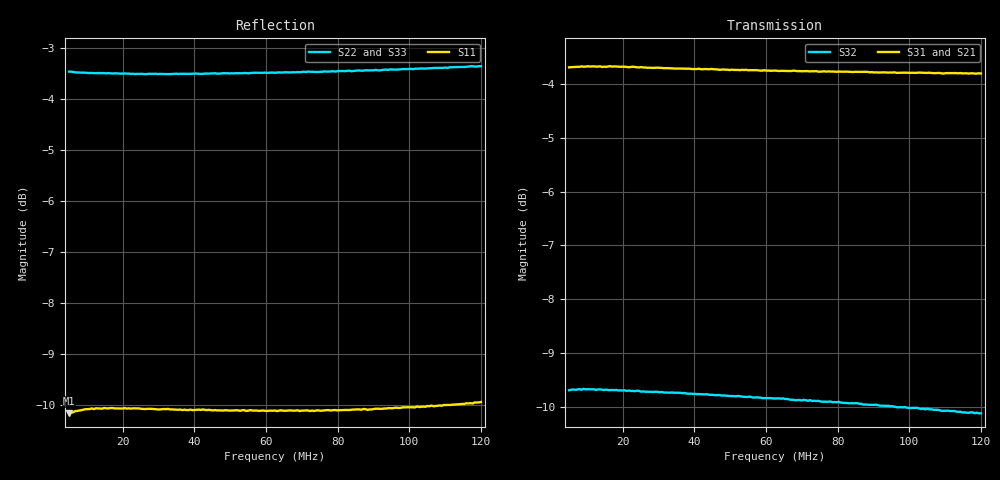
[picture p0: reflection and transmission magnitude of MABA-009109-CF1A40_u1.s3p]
#	MHz	S	RI	R	75
!FREQ	R1	I1	R2	I2	R3	I3
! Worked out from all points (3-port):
!   201 points, 5 MHz to 120 MHz, reference 75 ohm
!   strongest paths, dB at 5 MHz, 33.75 MHz, 62.5 MHz, 91.25 MHz, 120 MHz:
!     S31: -3.7, -3.7, -3.8, -3.8, -3.8
!     S21: -3.7, -3.7, -3.8, -4.0, -4.1
!     S32: -9.7, -9.7, -9.8, -10.0, -10.1
!   lowest |S11| = -10.2 dB at 5 MHz (marker M1), VSWR 1.90, Z = 142 + j2.55 ohm
!   |S11| at or under -10 dB: start of sweep to 109.5 MHz
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5  0.3104 0.00809  0.6537 -0.000275  -0.6537 -3.05e-05
   0.6537 -0.00104  -0.6712 0.00912  -0.3276 0.000549
   -0.6537 -3.05e-05  -0.3276 0.00061  -0.671 0.00891
6.725  0.3121 0.00117  0.6542 -0.00616  -0.6544 0.00583
       0.6542 -0.00607  -0.67 0.0103  -0.3284 0.00343
       -0.6544 0.00583  -0.3279 0.00288  -0.67 0.0094
10.75  0.3133 -0.0113  0.6545 -0.0154  -0.6547 0.015
       0.6548 -0.0154  -0.6689 0.0121  -0.3282 0.00797
       -0.6547 0.015  -0.3282 0.00772  -0.6685 0.0107
19.375  0.3124 -0.0312  0.6526 -0.0323  -0.6537 0.0311
        0.6523 -0.0327  -0.6678 0.0175  -0.3273 0.0165
        -0.6537 0.0311  -0.3271 0.0165  -0.6675 0.0145
33.75  0.3076 -0.0591  0.6481 -0.0573  -0.65 0.0558
       0.6481 -0.0577  -0.6672 0.0275  -0.3251 0.0289
       -0.65 0.0558  -0.3248 0.029  -0.6658 0.0228
62.5  0.2934 -0.1076  0.6349 -0.1035  -0.6412 0.1017
      0.6347 -0.1031  -0.6675 0.049  -0.3179 0.052
      -0.6412 0.1017  -0.3176 0.0522  -0.6628 0.0394
69.4  0.2888 -0.1181  0.6313 -0.1132  -0.639 0.1107
      0.6312 -0.1139  -0.668 0.0551  -0.316 0.0569
      -0.639 0.1107  -0.3157 0.057  -0.6624 0.044
71.7  0.2879 -0.1217  0.6297 -0.1167  -0.6381 0.1156
      0.6293 -0.1172  -0.6689 0.0572  -0.3153 0.059
      -0.6381 0.1156  -0.3148 0.0588  -0.6623 0.0455
88.375  0.2763 -0.1469  0.6202 -0.1416  -0.6321 0.1405
        0.6194 -0.142  -0.6693 0.07  -0.3099 0.0712
        -0.6321 0.1405  -0.3096 0.071  -0.6602 0.0547
120  0.2523 -0.1944  0.5965 -0.1848  -0.6178 0.1859
     0.5953 -0.1859  -0.6727 0.0957  -0.298 0.0916
     -0.6178 0.1859  -0.298 0.0918  -0.6568 0.071
